FUNCTION_BLOCK Preset_DUT

VAR_IN_OUT
    SD_SMD_IO: DUT_AMCI_Stepper;
END_VAR	

VAR_INPUT
	FB_Target_Position: DINT;
   		
END_VAR

VAR_OUTPUT
	Enable: BOOL :=FALSE;
	Error: BOOL :=TRUE;
END_VAR

VAR	
	I_Command_Word_1: UINT;
		
END_VAR

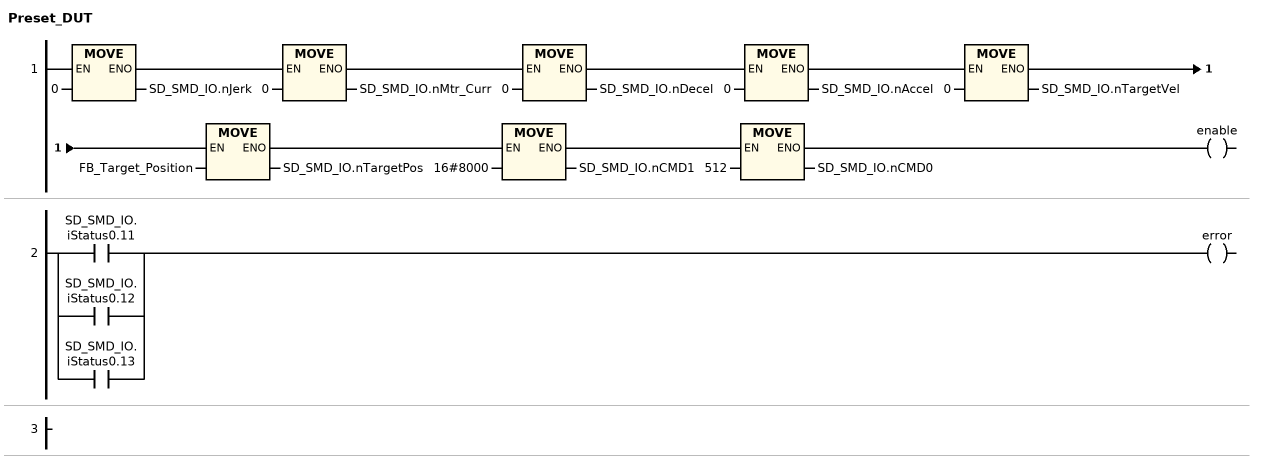
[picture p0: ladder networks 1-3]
// NETWORK 1
SD_SMD_IO.nJerk := 0;
SD_SMD_IO.nMtr_Curr := 0;
SD_SMD_IO.nDecel := 0;
SD_SMD_IO.nAccel := 0;
SD_SMD_IO.nTargetVel := 0;
SD_SMD_IO.nTargetPos := FB_Target_Position;
SD_SMD_IO.nCMD1 := 16#8000;
SD_SMD_IO.nCMD0 := 512;
enable := TRUE;

// NETWORK 2
error := SD_SMD_IO.iStatus0.11 OR SD_SMD_IO.iStatus0.12 OR SD_SMD_IO.iStatus0.13;

// NETWORK 3

END_FUNCTION_BLOCK
